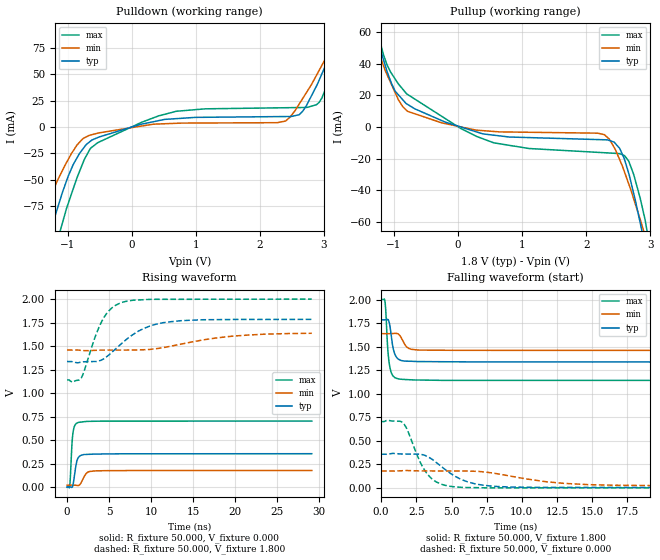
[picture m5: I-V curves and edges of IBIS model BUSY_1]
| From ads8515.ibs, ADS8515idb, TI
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|   BUSY OUTPUT Model  1.8V
[Model] BUSY_1
Model_type Output
Polarity   Non-Inverting
Enable   Active-Low
Vmeas = 0.9
Vref = 0.9
Cref = 15pF
Rref = 50
|   typ   min   max
|   typ   min   max
| AVERAGE
C_comp   7.39326E-12   6.3121E-12   7.6638E-12
| HIGH state
|C_comp   8.3783840e-12   7.3390870e-12   8.7297080e-12
| LOW state
|C_comp   6.0568170e-12   5.2851070e-12   6.9492180e-12
[Voltage Range]   1.8   1.65   2
[Temperature Range]   27   85   -40
[Pullup Reference]   1.8   1.65   2
[Pulldown Reference]   0   0   0
[Power Clamp Reference]   1.8   1.65   2
[GND Clamp Reference]   0   0   0
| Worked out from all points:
|   slope of the pulldown table from 0 to 0.27 V, typ, clamps not added: 64.2 ohm
|   slope of the pullup table from 0 to 0.27 V, typ, clamps not added: 78.7 ohm
|   falling waveform, R_fixture 50.000, V_fixture 1.800: 20-80 % time 313ps typ, 438ps min, 236ps max; typ from 1.78 V to 1.34 V
|   rising waveform, R_fixture 50.000, V_fixture 0.000: 20-80 % time 392ps typ, 594ps min, 273ps max; typ from 0.003 V to 0.356 V
|   rising waveform, R_fixture 50.000, V_fixture 1.800: 20-80 % time 4.11ns typ, 7.12ns min, 2.26ns max; typ from 1.34 V to 1.78 V
|   falling waveform, R_fixture 50.000, V_fixture 0.000: 20-80 % time 2.18ns typ, 4.2ns min, 1.31ns max; typ from 0.356 V to 0.003 V
[Pulldown]
|   Voltage   I(typ)   I(min)   I(max)
-1.8V     -217mA     -145.4mA   -308.8mA
-1.466V   -141.9mA   -93.68mA   -203.1mA
-1.217V   -88.79mA   -58.93mA   -127.1mA
-1.107V   -67.43mA   -44.66mA   -97.04mA
-910.9mV  -35.59mA   -22.57mA   -58.55mA
-663.1mV  -14.48mA   -8.02mA    -22.42mA
684.6mV   7.846mA    3.424mA    14.72mA
2.395V    9.876mA    5.531mA    18.24mA
2.663V    14.64mA    26.65mA    18.46mA
2.88V     38.57mA    48.81mA    21.09mA
3.27V     93.56mA    93.92mA    78.12mA
3.595V    141.2mA    132.6mA    139mA
[Pullup]
|   Voltage   I(typ)   I(min)   I(max)
-1.8V     132.4mA    111.5mA    160.2mA
-1.383V   71.95mA    62.53mA    82.26mA
-1.256V   54.75mA    48.71mA    59.99mA
-978.8mV  22.42mA    21.4mA     30.08mA
-786.7mV  14.21mA    9.849mA    20.49mA
552.1mV   -5.195mA   -2.844mA   -9.957mA
2.281V    -8.11mA    -4.875mA   -16.3mA
2.517V    -13.4mA    -20.37mA   -16.87mA
2.658V    -28.92mA   -35.68mA   -21.46mA
2.879V    -67.97mA   -63.73mA   -52.03mA
2.984V    -89.11mA   -78.25mA   -74.19mA
3.595V    -224.1mA   -172.9mA   -260.4mA
[Ramp]
R_load = 50
|   typ   min   max
dV/dt_r   0.216434/3.9044e-010   0.106789/5.88922e-010  0.426811/2.72131e-010
dV/dt_f   0.282363/3.0945e-010   0.116758/4.33921e-010  0.515694/2.34883e-010
[Falling Waveform]
R_fixture = 50.000
V_fixture = 1.800
V_fixture_min = 1.650
V_fixture_max = 2.000
C_fixture = 0.000
|  time   V(typ)   V(min)   V(max)
0s        1.785V     1.637V     2V
279.3ps   1.784V     1.637V     1.969V
338.4ps   1.786V     1.637V     1.85V
473.4ps   1.788V     1.637V     1.465V
637.5ps   1.703V     1.637V     1.266V
891.2ps   1.457V     1.639V     1.181V
1.238ns   1.365V     1.63V      1.156V
1.861ns   1.345V     1.49V      1.149V
2.628ns   1.341V     1.463V     1.145V
29.16ns   1.336V     1.459V     1.141V
[Rising Waveform]
R_fixture = 50.000
V_fixture = 0.000
V_fixture_min = 0.000
V_fixture_max = 0.000
C_fixture = 0.000
|  time   V(typ)   V(min)   V(max)
0s        2.996mV    22.28mV    -716.2uV
325.5ps   3.23mV     22.35mV    14.79mV
407.7ps   2.438mV    22.36mV    124.5mV
600.7ps   -655uV     22.4mV     473.5mV
753.5ps   43.85mV    22.43mV    602.7mV
1.141ns   266.7mV    20mV       680.5mV
1.352ns   316.4mV    18.83mV    689mV
2.353ns   348.8mV    152.2mV    700.1mV
3.251ns   352.4mV    173.2mV    701.4mV
29.16ns   356.4mV    178.3mV    703.5mV
[Rising Waveform]
R_fixture = 50.000
V_fixture = 1.800
V_fixture_min = 1.650
V_fixture_max = 2.000
C_fixture = 0.000
|  time   V(typ)   V(min)   V(max)
0s        1.336V     1.459V     1.141V
1.659ns   1.329V     1.455V     1.156V
3.371ns   1.337V     1.456V     1.603V
4.207ns   1.357V     1.458V     1.775V
5.224ns   1.425V     1.458V     1.897V
6.494ns   1.528V     1.458V     1.964V
9.157ns   1.689V     1.462V     1.994V
11.86ns   1.755V     1.491V     1.998V
19.69ns   1.784V     1.606V     1.999V
29.16ns   1.785V     1.637V     2V
[Falling Waveform]
R_fixture = 50.000
V_fixture = 0.000
V_fixture_min = 0.000
V_fixture_max = 0.000
C_fixture = 0.000
|  time   V(typ)   V(min)   V(max)
0s        356.4mV    178.3mV    703.5mV
1.547ns   358.8mV    181.6mV    690.5mV
2.768ns   355.7mV    179.2mV    274.5mV
3.222ns   336.5mV    179.1mV    158mV
3.896ns   271.1mV    179mV      64.31mV
4.836ns   163mV      178.8mV    17.24mV
6.145ns   63.05mV    178.1mV    3.098mV
8.094ns   14.94mV    153.2mV    -182uV
14.68ns   3.726mV    33.92mV    -349.1uV
29.16ns   2.996mV    22.28mV    -716.2uV
